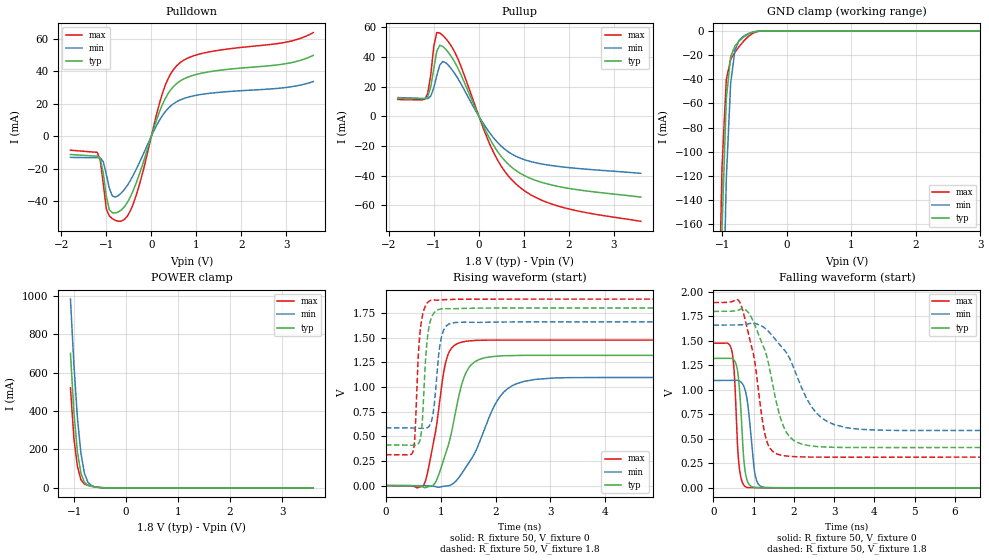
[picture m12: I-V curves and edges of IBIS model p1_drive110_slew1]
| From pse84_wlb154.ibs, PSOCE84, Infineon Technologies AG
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[Model] p1_drive110_slew1
Model_type I/O
Polarity  Non-Inverting
Enable   Active-High
Vinl  =  0.54
Vinh  =  1.26
Vmeas =  0.9
Cref  =  15pF
| Capacitance   typ   min   max
C_comp   1.187163e-12   1.148471e-12   1.233738e-12
| Variables   typ   min   max
[GND Clamp Reference]   0   0   0
[POWER Clamp Reference]   1.8   1.66   1.89
[Pulldown Reference]   0   0   0
[Pullup Reference]   1.8   1.66   1.89
[Temperature Range]   25   125   -40
[Voltage Range]   1.8   1.66   1.89
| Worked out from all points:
|   slope of the pulldown table from 0 to 0.27 V, typ, clamps not added: 12.9 ohm
|   slope of the pullup table from 0 to 0.27 V, typ, clamps not added: 16.3 ohm
|   GND clamp passes 1 mA (typ) near -0.51 V on its own axis
|   POWER clamp passes 1 mA (typ) near -0.47 V on its own axis
|   rising waveform, R_fixture 50, V_fixture 0: 20-80 % time 345ps typ, 550ps min, 246ps max; typ from 0 V to 1.32 V
|   rising waveform, R_fixture 50, V_fixture 1.8: 20-80 % time 94.3ps typ, 114ps min, 86.1ps max; typ from 0.411 V to 1.8 V
|   falling waveform, R_fixture 50, V_fixture 0: 20-80 % time 123ps typ, 158ps min, 105ps max; typ from 1.32 V to 0 V
|   falling waveform, R_fixture 50, V_fixture 1.8: 20-80 % time 526ps typ, 809ps min, 373ps max; typ from 1.8 V to 0.411 V
[GND Clamp]
| Voltage   I(typ)   I(min)   I(max)
-1.137V   -618.8mA   -753.3mA   -532.4mA
-1.07V    -360.9mA   -497.6mA   -281.1mA
-1.003V   -163.7mA   -277.5mA   -113mA
-936.6mV  -56.21mA   -122.2mA   -40.06mA
-869.7mV  -21.33mA   -43.29mA   -23.66mA
-802.8mV  -12.5mA    -15.96mA   -17.71mA
-735.9mV  -8.345mA   -7.674mA   -12.88mA
-669mV    -5.267mA   -4.349mA   -8.574mA
-535.2mV  -1.314mA   -1.207mA   -2.328mA
-401.4mV  -73.55uA   -132.2uA   -119.3uA
3.6V      0A         0A         0A
[POWER Clamp]
| Voltage   I(typ)   I(min)   I(max)
-1.07V    700.8mA    983.4mA    521.5mA
-1.003V   391.6mA    640.4mA    255.8mA
-936.6mV  187.6mA    365.2mA    112.5mA
-869.7mV  77.29mA    181mA      42.73mA
-802.8mV  28.91mA    77.52mA    19.98mA
-735.9mV  13.13mA    29.19mA    13.35mA
-669mV    7.755mA    11.55mA    8.955mA
-535.2mV  2.356mA    2.862mA    2.667mA
-334.5mV  34.33uA    127.4uA    15.58uA
3.6V      0A         0A         0A
[Pullup]
| Voltage   I(typ)   I(min)   I(max)
-1.8V     12.09mA    12.65mA    11.3mA
-1.204V   11.78mA    11.99mA    11.48mA
-1.07V    19.86mA    13.72mA    28.2mA
-1.003V   32.33mA    19.19mA    47.33mA
-936.6mV  43.91mA    27.54mA    56.42mA
-869.7mV  47.86mA    34.63mA    56.15mA
-735.9mV  45.08mA    36.1mA     52.32mA
-468.3mV  32.54mA    25.54mA    38.83mA
310.3mV   -18.74mA   -13.89mA   -23.34mA
806.9mV   -36.12mA   -26.64mA   -45.07mA
1.738V    -47.05mA   -33.63mA   -60.21mA
3.6V      -54.39mA   -38.4mA    -70.69mA
[Pulldown]
| Voltage   I(typ)   I(min)   I(max)
-1.8V     -11.32mA   -13.07mA   -8.649mA
-1.204V   -12.34mA   -13.28mA   -9.975mA
-1.137V   -13.74mA   -13.28mA   -14.92mA
-1.003V   -36.81mA   -23.32mA   -44.61mA
-936.6mV  -45.26mA   -32.01mA   -49.07mA
-869.7mV  -47.16mA   -36.77mA   -50.78mA
-669mV    -45.45mA   -34.98mA   -52.27mA
-401.4mV  -33.26mA   -23.95mA   -41.52mA
248.3mV   19.63mA    12.78mA    26.5mA
558.6mV   32.22mA    21.08mA    43.15mA
1.117V    38.7mA     25.67mA    50.79mA
3.6V      49.63mA    33.56mA    63.68mA
[Ramp]
dV/dt_r   0.792036/0.345492n  0.657068/0.550083n  0.88488/0.246133n
dV/dt_f   0.833231/0.526279n  0.644607/0.809114n  0.946072/0.372778n
R_load = 50
[Rising Waveform]
R_fixture = 50
V_fixture = 0
V_fixture_min = 0
V_fixture_max = 0
| Time   V(typ)   V(min)   V(max)
0s        11.49nV    820.1nV    4.137nV
678ps     -12.81mV   -22.99uV   -1.954mV
887.1ps   18.51mV    -7.51mV    489mV
1.045ns   246mV      -7.364mV   1.116V
1.128ns   389.5mV    -2.363mV   1.32V
1.388ns   1.034V     126.1mV    1.454V
1.614ns   1.252V     322.4mV    1.471V
2.145ns   1.316V     945.3mV    1.475V
3.069ns   1.32V      1.091V     1.475V
50ns      1.32V      1.095V     1.475V
[Rising Waveform]
R_fixture = 50
V_fixture = 1.8
V_fixture_min = 1.66
V_fixture_max = 1.89
| Time   V(typ)   V(min)   V(max)
0s        411.3mV    585.7mV    313.2mV
500.8ps   407.9mV    583.1mV    355.2mV
532.1ps   407.9mV    582mV      521.5mV
619.2ps   453.8mV    579.9mV    1.531V
662.4ps   631.7mV    579.2mV    1.71V
748.8ps   1.45V      583.7mV    1.847V
856ps     1.731V     714.5mV    1.881V
1.022ns   1.792V     1.524V     1.883V
1.338ns   1.795V     1.655V     1.889V
50ns      1.8V       1.66V      1.89V
[Falling Waveform]
R_fixture = 50
V_fixture = 0
V_fixture_min = 0
V_fixture_max = 0
| Time   V(typ)   V(min)   V(max)
0s        1.32V      1.095V     1.475V
447.3ps   1.32V      1.096V     1.418V
514.2ps   1.302V     1.097V     1.202V
569.9ps   1.253V     1.097V     711.6mV
666.9ps   910.2mV    1.086V     141mV
769.6ps   234.8mV    1.023V     20.86mV
878.6ps   41.09mV    770.6mV    2.404mV
1.063ns   2.842mV    89.9mV     2.737mV
1.355ns   2.561mV    2.603mV    865.2uV
50ns      11.46nV    829.7nV    4.141nV
[Falling Waveform]
R_fixture = 50
V_fixture = 1.8
V_fixture_min = 1.66
V_fixture_max = 1.89
| Time   V(typ)   V(min)   V(max)
0s        1.8V       1.66V      1.89V
617.8ps   1.812V     1.661V     1.915V
904.7ps   1.768V     1.676V     1.515V
1.231ns   1.453V     1.644V     655.7mV
1.357ns   1.292V     1.6V       441.4mV
1.66ns    722mV      1.455V     335.6mV
1.962ns   495.9mV    1.26V      319mV
2.684ns   418.1mV    716.2mV    313.2mV
4.059ns   411mV      588.9mV    313.2mV
50ns      411.3mV    585.7mV    313.2mV
